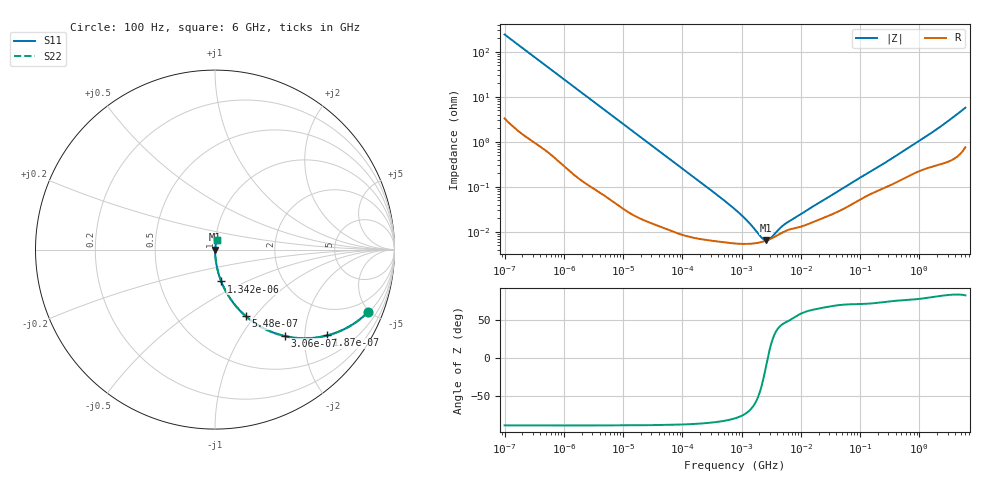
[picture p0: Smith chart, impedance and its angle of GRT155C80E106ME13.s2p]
!Murata Part Number: GRT155C80E106ME13
!These Parameters are Measured in Series Mode Connection
!Data Generated on Jun 19, 2026
!  o--ll--o
!Port1  Port2
!  o------o
!Operation Temp=25[degC], DC Bias Voltage=0[V]
!Freq. Start=100[Hz] Stop=6[GHz] 401[Steps]
# Hz S RI R 50
!Freq.(Hz) S11(Real) S11(Imag) S21(Real) S21(Imag) S12(Real) S12(Imag) S22(Real) S22(Imag)
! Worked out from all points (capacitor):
!   401 points, 100 Hz to 6 GHz, reference 50 ohm
!   read as one part in series: C = 6.55 uF near 109 Hz
!   lowest |Z| = 6.45 mohm at 2.595 MHz (marker M1)
!   series resonance near 2.773 MHz, so ESL is about 500 pH
!   S11 on the Smith chart (normalised r, x): 100 Hz: 1.07, -4.85; 187 Hz: 1.03, -2.60; 306 Hz: 1.02, -1.59; 548 Hz: 1.01, -0.89; 1.342 kHz: 1.00, -0.37; 6 GHz: 1.02, +0.11
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100  0.8512 -0.3492  0.1488 0.3492  0.1488 0.3492  0.8512 -0.3492
131  0.7721 -0.4132  0.2279 0.4132  0.2279 0.4132  0.7721 -0.4132
187  0.6266 -0.4777  0.3734 0.4777  0.3734 0.4777  0.6266 -0.4777
306  0.3896 -0.4815  0.6104 0.4815  0.6104 0.4815  0.3896 -0.4815
548  0.17 -0.3693  0.83 0.3693  0.83 0.3693  0.17 -0.3693
820  0.0854 -0.2735  0.9146 0.2735  0.9146 0.2735  0.0854 -0.2735
1342  0.0346 -0.1773  0.9654 0.1773  0.9654 0.1773  0.0346 -0.1773
2008  0.0163 -0.1211  0.9837 0.1211  0.9837 0.1211  0.0163 -0.1211
6433  0.00199 -0.0387  0.998 0.0387  0.998 0.0387  0.00199 -0.0387
40335  0.000172 -0.00626  0.9998 0.00626  0.9998 0.00626  0.000172 -0.00626
345986  6.26e-05 -0.000734  0.9999 0.000734  0.9999 0.000734  6.26e-05 -0.000734
774597  5.48e-05 -0.00031  0.9999 0.00031  0.9999 0.00031  5.48e-05 -0.00031
1159002  5.37e-05 -0.000186  0.9999 0.000186  0.9999 0.000186  5.37e-05 -0.000186
1734173  5.57e-05 -9.1e-05  0.9999 9.1e-05  0.9999 9.1e-05  5.57e-05 -9.1e-05
1983483  5.75e-05 -6.34e-05  0.9999 6.34e-05  0.9999 6.34e-05  5.75e-05 -6.34e-05
2594782  6.34e-05 -1.21e-05  0.9999 1.21e-05  0.9999 1.21e-05  6.34e-05 -1.21e-05
3882480  8.11e-05 5.83e-05  0.9999 -5.83e-05  0.9999 -5.83e-05  8.11e-05 5.83e-05
5809218  0.000107 0.000117  0.9999 -0.000117  0.9999 -0.000117  0.000107 0.000117
1.555665e7  0.000161 0.000318  0.9998 -0.000318  0.9998 -0.000318  0.000161 0.000318
3.124326e8  0.00107 0.00377  0.9989 -0.00377  0.9989 -0.00377  0.00107 0.00377
1.637704e9  0.00302 0.0157  0.997 -0.0157  0.997 -0.0157  0.00302 0.0157
6e9  0.0106 0.0557  0.9894 -0.0557  0.9894 -0.0557  0.0106 0.0557
